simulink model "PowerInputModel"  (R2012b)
settings: Solver=ode45  StartTime=0.0  StopTime=50  RelTol=1e-3
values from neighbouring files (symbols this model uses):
  Ct = 2700    [PowerInputValidationTest.m]    (also in SimulationScript.m; SCmodel.m)
  Imax = 2*Q/3600    (= 4)    [PowerInputValidationTest.m]
  Imin = 5*Q/3600    (= 10)    [PowerInputValidationTest.m]
  Ki = 0.8    [PowerInputValidationTest.m]
  Kp = 2    [PowerInputValidationTest.m]
  Q = 2*3600    (= 7200)    [PowerInputValidationTest.m]    (also in SimulationScript.m; SCmodel.m)
  Rs = 0.008    [PowerInputValidationTest.m]    (also in SimulationScript.m; SCmodel.m)
  Rt = 0.011    [PowerInputValidationTest.m]    (also in SimulationScript.m; SCmodel.m)
  SOC = [0 0.1 0.2 0.3 0.4 0.5 0.6 0.7 0.8 0.9 1]    [PowerInputValidationTest.m]    (also in SimulationScript.m; SCmodel.m; int_series.m = 1:1:101)
  SOC_0 = 0.5    [PowerInputValidationTest.m]    (also in SimulationScript.m; SCmodel.m)
  V = [2.25 3.2 3.25 3.25 3.3 3.3 3.3 3.35 3.35 3.35 3.75]    [PowerInputValidationTest.m]    (also in SimulationScript.m; SCmodel.m; int_series.m = [2.000; 2.760; 2.885; 2.963; 3.020; 3.066; 3.103; 3.136; 3.1)
undefined symbols (not defined in the file or in its folder): InitialSOC

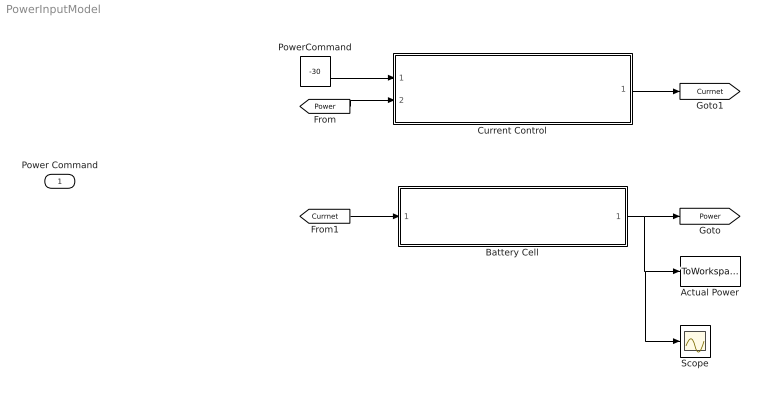
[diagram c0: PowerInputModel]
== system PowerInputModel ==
  Power Command : Inport
  Actual Power : ToWorkspace  VariableName=actualpower  SampleTime=-1  SaveFormat=Structure With Time
  Battery Cell : Subsystem
  Current Control : Subsystem
  PowerCommand : Constant  Value=-30
  Scope : Scope
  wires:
  Battery Cell/1("outputpower, Watt") -> [Power], Scope/1, Actual Power/1
  [Power] -> Current Control/2(Actual Power [w])
  PowerCommand/1 -> Current Control/1(Power Command [w])
  Current Control/1(PI Current message [A]) -> [Currnet]
  [Currnet] -> Battery Cell/1(In1)

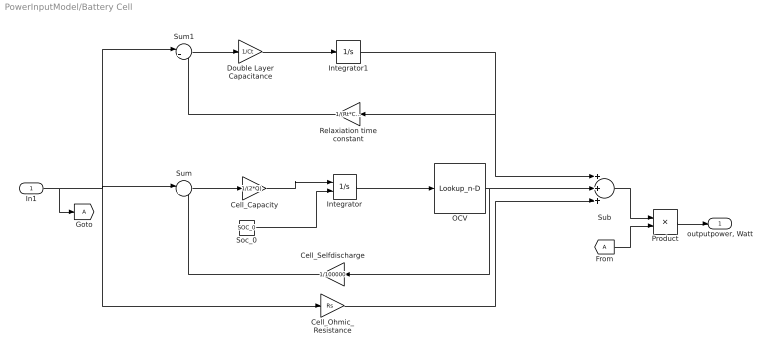
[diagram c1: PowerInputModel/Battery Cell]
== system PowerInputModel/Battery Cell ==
  In1 : Inport
  Cell_Capacity : Gain  Gain=1/(2*Q)
  Cell_Ohmic_Resistance : Gain  Gain=Rs
  Cell_Selfdischarge : Gain  Gain=1/100000
  Double Layer Capacitance : Gain  Gain=1/Ct
  From : From
  Integrator : Integrator  InitialConditionSource=external  InitialCondition=InitialSOC
  Integrator1 : Integrator
  OCV : Lookup_n-D  NumberOfTableDimensions=1  BreakpointsForDimension1=SOC  Table=V  RndMeth=Simplest
  Product : Product
  Relaxiation time constant : Gain  Gain=1/(Rt*Ct)
  Soc_0 : Constant  Value=SOC_0
  Sub : Sum  Inputs=+++
  Sum : Sum  Inputs=|+-
  Sum1 : Sum  Inputs=|+-
  "outputpower, Watt" : Outport
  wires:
  Integrator/1 -> OCV/1
  OCV/1 -> Cell_Selfdischarge/1, Sub/2
  In1/1 -> [A], Sum1/1, Cell_Ohmic_Resistance/1, Sum/1
  Cell_Capacity/1 -> Integrator/1
  Cell_Selfdischarge/1 -> Sum/2
  Integrator1/1 -> Relaxiation time constant/1, Sub/1
  Relaxiation time constant/1 -> Sum1/2
  Cell_Ohmic_Resistance/1 -> Sub/3
  Sum/1 -> Cell_Capacity/1
  Double Layer Capacitance/1 -> Integrator1/1
  Sum1/1 -> Double Layer Capacitance/1
  Soc_0/1 -> Integrator/2
  Sub/1 -> Product/1
  From/1 -> Product/2
  Product/1 -> "outputpower, Watt"/1

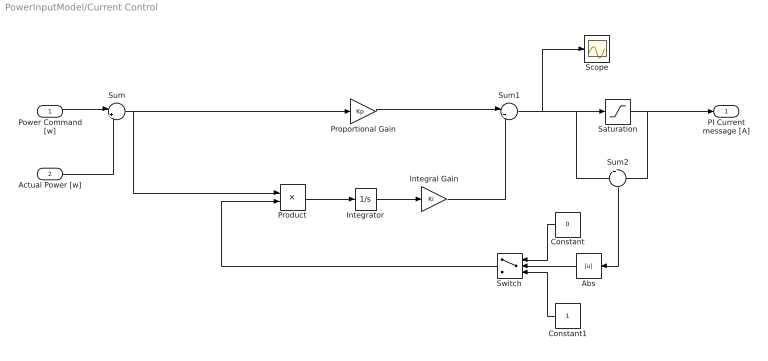
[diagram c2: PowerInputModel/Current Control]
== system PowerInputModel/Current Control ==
  Power Command [w] : Inport
  Actual Power [w] : Inport  Port=2
  Abs : Abs
  Constant : Constant  Value=0
  Constant1 : Constant
  Integrator : Integrator
  Product : Product
  Proportional Gain : Gain  Gain=Kp
  Saturation : Saturate  UpperLimit=Imax  LowerLimit=-Imin  ZeroCross=off
  Scope : Scope
  Sum : Sum  Inputs=|+-
  Sum1 : Sum  Inputs=|++
  Sum2 : Sum  Inputs=+-
  Switch : Switch  Threshold=0.01  ZeroCross=off
  lntegral Gain : Gain  Gain=Ki
  PI Current message [A] : Outport
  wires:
  Power Command [w]/1 -> Sum/1
  Actual Power [w]/1 -> Sum/2
  Sum/1 -> Proportional Gain/1, Product/1
  Proportional Gain/1 -> Sum1/1
  Sum1/1 -> Scope/1, Saturation/1, Sum2/1
  Saturation/1 -> PI Current message [A]/1, Sum2/2
  Integrator/1 -> lntegral Gain/1
  lntegral Gain/1 -> Sum1/2
  Sum2/1 -> Abs/1
  Abs/1 -> Switch/2
  Constant/1 -> Switch/1
  Constant1/1 -> Switch/3
  Switch/1 -> Product/2
  Product/1 -> Integrator/1
